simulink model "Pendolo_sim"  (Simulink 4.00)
settings: Solver=ode45  StartTime=0.0  StopTime=10.0  RelTol=1e-3
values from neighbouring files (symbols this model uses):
  csi = 0.05    [pendolo.m]
  lambda = 0.5    [pendolo.m]
  w = r*w0    [pendolo.m]
  w0 = sqrt(9.81/L)    [pendolo.m]
  x0 = 0    [pendolo.m]
  xp0 = 0    [pendolo.m]

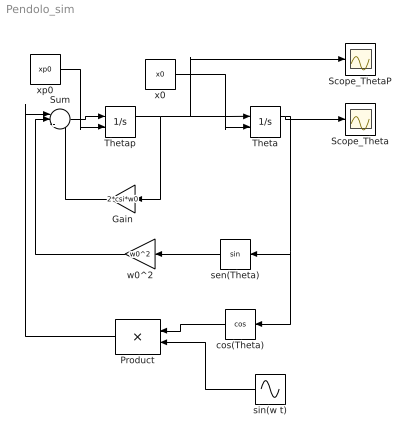
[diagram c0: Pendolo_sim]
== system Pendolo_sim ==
  Gain : Gain  Orientation=left  Gain=2*csi*w0  Multiplication=Element-wise(K.*u)  SaturateOnIntegerOverflow=on
  Product : Product  Orientation=left  Inputs=2  Multiplication=Element-wise(.*)  SaturateOnIntegerOverflow=on
  Scope_Theta : Scope
  Scope_ThetaP : Scope
  Sum : Sum  Inputs=|+--  SaturateOnIntegerOverflow=on
  Theta : Integrator  ExternalReset=none  InitialConditionSource=external  InitialCondition=0  LimitOutput=off  UpperSaturationLimit=inf  LowerSaturationLimit=-inf  ShowSaturationPort=off  ShowStatePort=off  AbsoluteTolerance=auto
  Thetap : Integrator  ExternalReset=none  InitialConditionSource=external  InitialCondition=0  LimitOutput=off  UpperSaturationLimit=inf  LowerSaturationLimit=-inf  ShowSaturationPort=off  ShowStatePort=off  AbsoluteTolerance=auto
  cos(Theta) : Trigonometry  Orientation=left  Operator=cos  OutputSignalType=auto
  sen(Theta) : Trigonometry  Orientation=left  Operator=sin  OutputSignalType=auto
  sin(w t) : Sin  Orientation=left  SineType=Time-based  Amplitude=w^2*lambda  Bias=0  Frequency=w  Phase=0  Samples=10  SampleTime=0
  w0^2 : Gain  Orientation=left  Gain=w0^2  Multiplication=Element-wise(K.*u)  SaturateOnIntegerOverflow=on
  x0 : Constant  Value=x0
  xp0 : Constant  Value=xp0
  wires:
  Thetap/1 -> Gain/1, Theta/1, Scope_ThetaP/1
  Sum/1 -> Thetap/1
  Gain/1 -> Sum/3
  Theta/1 -> sen(Theta)/1, cos(Theta)/1, Scope_Theta/1
  sen(Theta)/1 -> w0^2/1
  w0^2/1 -> Sum/2
  cos(Theta)/1 -> Product/1
  sin(w t)/1 -> Product/2
  Product/1 -> Sum/1
  xp0/1 -> Thetap/2
  x0/1 -> Theta/2
